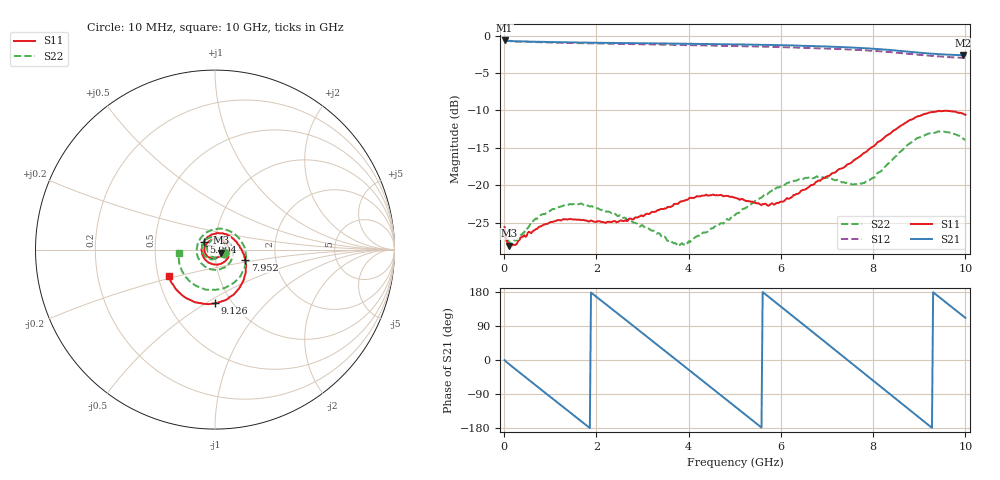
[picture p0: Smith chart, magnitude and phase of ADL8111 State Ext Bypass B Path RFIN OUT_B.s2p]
! Analog Devices Inc.
! Device:  ADL8111
! Description: Bypass Amplifier
! Frequency:  0.00 -  8.00 GHz
! Package:28-Lead Lead Frame Chip Scale Package[LFCSP] 6mm by 6mm
! Conditions:	Vdd = 5.0 V
!		State: External Bypass A
!		Path:  RFIN (Port1) to OUT_B (Port 2)
!		Idq = 70mA
!		Pin = -10 dBm
!		Temp = +25 C (baseplate temperature)
! Freq(Hz)	S11a(dB)	S11p(deg)	S21a(dB)	S21p(deg)	S12a(dB)	S12p(deg)	S22a(dB)	S22p(deg)
# Hz S  dB  R 50
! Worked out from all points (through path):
!   401 points, 10 MHz to 10 GHz, reference 50 ohm
!   highest |S21| = -0.65 dB at 10 MHz (marker M1); lowest = -2.6 dB at 9.95 GHz (marker M2)
!   group delay of S21, straight-line fit = 269 ps
!   lowest |S11| = -28.1 dB at 109.9 MHz (marker M3), VSWR 1.08, Z = 53.6 - j1.92 ohm
!   |S11| at or under -10 dB: start of sweep to end of sweep
!   |S22| runs from -28.2 to -12.8 dB; largest |S21 - S12| = 0.03
!   S11 on the Smith chart (normalised r, x): 10 MHz: 1.10, -0.05; 5.904 GHz: 0.88, +0.07; 7.952 GHz: 1.40, -0.16; 9.126 GHz: 0.84, -0.55; 10 GHz: 0.57, -0.18
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1e7  -25.62 -23.6  -0.65 -0.3  -0.66 -0.6  -25.92 -19.6
1.099e8  -28.08 -26.9  -0.72 -11.2  -0.72 -11.1  -27.74 -26.6
8.84125e8  -25.24 -126.8  -0.85 -86.0  -0.91 -86.0  -23.89 -139.6
1.25875e9  -24.64 -164.6  -0.89 -122.0  -0.97 -122.0  -22.81 176.1
1.683325e9  -24.67 158.0  -0.94 -162.8  -1.02 -162.8  -22.48 130.2
2.1079e9  -24.93 130.4  -0.96 156.5  -1.06 156.5  -23.35 81.5
2.6074e9  -24.77 97.9  -1.01 108.5  -1.12 108.5  -24.35 22.8
2.95705e9  -24.11 75.2  -1.03 74.9  -1.16 74.9  -25.52 -22.0
3.35665e9  -23.35 46.9  -1.06 36.4  -1.20 36.4  -26.44 -74.6
4.030975e9  -21.67 -3.7  -1.10 -28.6  -1.27 -28.6  -27.61 -174.8
4.530475e9  -21.27 -49.6  -1.14 -76.7  -1.33 -76.8  -25.78 124.5
5.005e9  -21.70 -98.9  -1.18 -122.6  -1.40 -122.6  -24.00 80.3
5.45455e9  -22.39 -153.2  -1.23 -166.2  -1.46 -166.1  -22.09 46.9
5.9041e9  -22.41 147.5  -1.27 150.2  -1.53 150.2  -20.34 10.6
6.3037e9  -21.33 99.6  -1.34 111.3  -1.60 111.4  -19.40 -27.2
6.678325e9  -19.99 62.7  -1.40 74.9  -1.68 74.9  -19.08 -66.7
7.327675e9  -17.75 15.5  -1.55 11.5  -1.82 11.5  -19.64 -151.0
7.95205e9  -15.00 -18.2  -1.74 -49.8  -2.03 -49.8  -19.18 101.8
8.35165e9  -13.16 -40.8  -1.91 -89.1  -2.20 -89.1  -17.01 35.8
9.125875e9  -10.47 -89.8  -2.35 -164.5  -2.64 -164.5  -13.30 -68.9
9.95005e9  -10.45 -147.1  -2.63 116.1  -2.98 116.1  -13.78 -168.2
1e10  -10.60 -150.6  -2.62 111.2  -2.97 111.2  -13.95 -175.1
